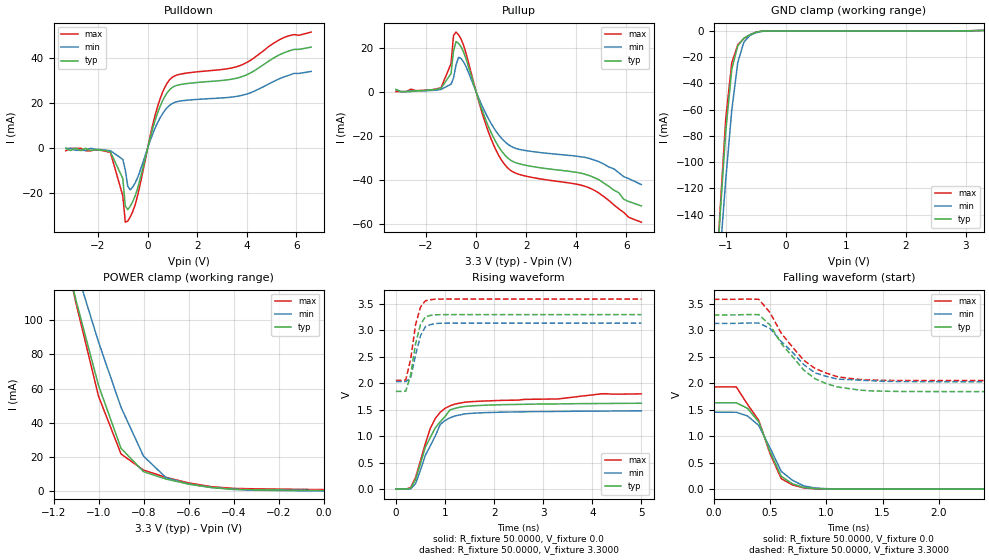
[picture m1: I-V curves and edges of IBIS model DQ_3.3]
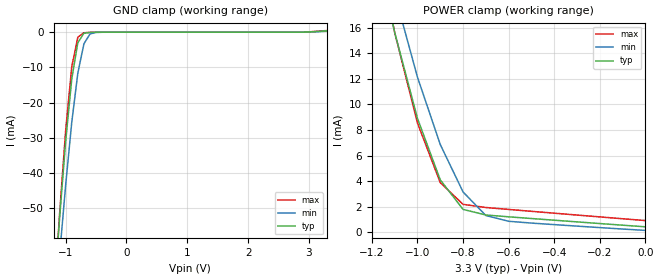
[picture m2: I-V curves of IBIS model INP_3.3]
|*** ISSI Synchronous Sram IBIS Model ***
[IBIS ver]	3.2
[File name]	is61lf204836b100tq.ibs
[File Rev]	1.0
[Date]	May 13,2013
[Notes]
|--- Version History --------------------------------
|1.0: prelimiary
[Disclaimer]	This information is for modeling purpose only
		and is not guaranteed
[Copyright]	INTEGRATED SILICON SOLUTION, INC. 2011
[Component]	IS61LF204836B_100TQ
[Manufacturer]	ISSI
[Package]
| variable   typ   min   max
R_pkg		105.88m			21.330m			174.58m
L_pkg		1.8700nH		0.5900nH		2.5200nH
C_pkg		0.2100pF		0.0600pF		0.2800pF
[Pin]  signal_name   model_name   R_pin   L_pin   C_pin
100   A   INP_3.3
99   A   INP_3.3
98   CEB   INP_3.3
97   CE2   INP_3.3
96   NC   NC
95   NC   NC
94   BWbB   INP_3.3
93   BWaB   INP_3.3
92   CE2B   INP_3.3
91   VDD   POWER
90   VSS   GND
89   CLK   INP_3.3
88   GWB   INP_3.3
87   BWEB   INP_3.3
86   OEB   INP_3.3
85   ADSCB   INP_3.3
84   ADSPB   INP_3.3
83   ADVB   INP_3.3
82   A   INP_3.3
81   A   INP_3.3
80   DQPb   DQ_3.3
79   DQb   DQ_3.3
78   DQb   DQ_3.3
77   VDDQ   POWER
76   VSS   GND
75   DQb   DQ_3.3
74   DQb   DQ_3.3
73   DQb   DQ_3.3
72   DQb   DQ_3.3
71   VSS   GND
70   VDDQ   POWER
69   DQb   DQ_3.3
68   DQb   DQ_3.3
67   VSS   GND
66   NC   NC
65   VDD   POWER
64   ZZ   INP_3.3
63   DQa   DQ_3.3
62   DQa   DQ_3.3
61   VDDQ   POWER
60   VSS   GND
59   DQa   DQ_3.3
58   DQa   DQ_3.3
57   DQa   DQ_3.3
56   DQa   DQ_3.3
55   VSS   GND
54   VDDQ   POWER
53   DQa   DQ_3.3
52   DQa   DQ_3.3
51   DQPa   DQ_3.3
50   A   INP_3.3
49   A   INP_3.3
48   A   INP_3.3
47   A   INP_3.3
46   A   INP_3.3
45   A   INP_3.3
44   A   INP_3.3
43   A   INP_3.3
42   A   INP_3.3
41   VDD   POWER
40   VSS   GND
39   A   INP_3.3
38   A   INP_3.3
37   A0   INP_3.3
36   A1   INP_3.3
35   A   INP_3.3
34   A   INP_3.3
33   A   INP_3.3
32   A   INP_3.3
31   MODE   INP_3.3
30   DQPd   DQ_3.3
29   DQd   DQ_3.3
28   DQd   DQ_3.3
27   VDDQ   POWER
26   VSS   GND
25   DQd   DQ_3.3
24   DQd   DQ_3.3
23   DQd   DQ_3.3
22   DQd   DQ_3.3
21   VSS   GND
20   VDDQ   POWER
19   DQd   DQ_3.3
18   DQd   DQ_3.3
17   VSS   GND
16   NC   NC
15   VDD   POWER
14   NC   NC
13   DQc   DQ_3.3
12   DQc   DQ_3.3
11   VDDQ   POWER
10   VSS   GND
9   DQc   DQ_3.3
8   DQc   DQ_3.3
7   DQc   DQ_3.3
6   DQc   DQ_3.3
5   VSS   GND
4   VDDQ   POWER
3   DQc   DQ_3.3
2   DQc   DQ_3.3
1   DQPc   DQ_3.3
| Models and submodels in the file (2): DQ_3.3 (3-state), INP_3.3 (Input)
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|   Model DQ_3.3
[Model]		DQ_3.3
Model_type	3-state
Polarity   Non-Inverting
Enable   Active-Low
Vmeas = 	0.7500V
Cref = 		5.0000pF
Rref = 		50.0000
Vref = 		1.2500V
C_comp   3.8290pF   3.3420pF   4.0300pF|
[Temperature Range]	  25.0000   100.0000   0.0
[Voltage Range]   3.3000V   3.1350V   3.6000V
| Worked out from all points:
|   slope of the pulldown table from 0 to 0.495 V, typ, clamps not added: 26.9 ohm
|   slope of the pullup table from 0 to 0.495 V, typ, clamps not added: 31.2 ohm
|   GND clamp passes 1 mA (typ) near -0.49 V on its own axis
|   POWER clamp passes 1 mA (typ) near -0.36 V on its own axis
|   rising waveform, R_fixture 50.0000, V_fixture 0.0: 20-80 % time 480ps typ, 408ps min, 447ps max; typ from 0 V to 1.62 V
|   rising waveform, R_fixture 50.0000, V_fixture 3.3000: 20-80 % time 178ps typ, 175ps min, 176ps max; typ from 1.84 V to 3.29 V
|   falling waveform, R_fixture 50.0000, V_fixture 0.0: 20-80 % time 195ps typ, 217ps min, 242ps max; typ from 1.63 V to 0 V
|   falling waveform, R_fixture 50.0000, V_fixture 3.3000: 20-80 % time 343ps typ, 315ps min, 335ps max; typ from 3.29 V to 1.84 V
[Pulldown]
|Voltage	  I(typ)   I(min)   I(max)
-3.3V     0A         0A         -1.1mA
-1.5V     -1.6mA     -1.08mA    -1.87mA
-1V       -13.48mA   -4.95mA    -21.15mA
-900mV    -25.69mA   -9.639mA   -32.88mA
-800mV    -27.28mA   -16.91mA   -32.39mA
-700mV    -25.77mA   -18.5mA    -30.54mA
-500mV    -21.13mA   -15.36mA   -25.04mA
400mV     15.63mA    11.35mA    18.49mA
900mV     26.18mA    19.21mA    30.66mA
3.7V      31.51mA    23.31mA    36.7mA
5.5V      42.5mA     31.77mA    49.28mA
6.6V      45mA       34.2mA     51.7mA
[Pullup]
|Voltage	  I(typ)   I(min)   I(max)
-3.2V     1mA        900uA      0A
-1.4V     1.5mA      990uA      1.76mA
-1V       8.19mA     3.366mA    12.71mA
-900mV    18.53mA    6.147mA    25.54mA
-800mV    22.75mA    12.11mA    27.08mA
-700mV    21.98mA    15.63mA    25.89mA
-500mV    18.06mA    13.53mA    21.17mA
400mV     -13.22mA   -10.27mA   -15.35mA
1.2V      -29.47mA   -23.28mA   -33.95mA
1.9V      -33.32mA   -26.66mA   -38.21mA
4.5V      -38.1mA    -30.33mA   -43.68mA
6.6V      -52mA      -42.3mA    -59.4mA
[GND_clamp]
|Voltage	  I(typ)   I(min)   I(max)
-3.3V     -1.893A    -1.626A    -2.116A
-1.2V     -220.2mA   -237.3mA   -225.5mA
-1.1V     -144.4mA   -173.5mA   -140.5mA
-1V       -76.37mA   -113.2mA   -66.76mA
-900mV    -29.2mA    -60.35mA   -24.24mA
-800mV    -11.34mA   -23.99mA   -10.52mA
-700mV    -5.573mA   -8.7mA     -5.892mA
-600mV    -2.907mA   -3.457mA   -3.011mA
-500mV    -1.075mA   -1.407mA   -999.8uA
-300mV    -9.492uA   -41.34uA   -5.052uA
3.3V      423.1uA    322.6uA    488.5uA
[POWER_clamp]
|Voltage	  I(typ)   I(min)   I(max)
-3.3V     1.424A     1.197A     1.604A
-1.2V     166.3mA    175.1mA    171.7mA
-1.1V     111.5mA    129.9mA    109.8mA
-1V       61.82mA    87.17mA    55.51mA
-900mV    25.05mA    49.03mA    21.74mA
-800mV    11.41mA    20.46mA    12.33mA
-700mV    7.064mA    7.924mA    8.056mA
-600mV    4.166mA    4.141mA    4.82mA
-500mV    2.143mA    2.162mA    2.625mA
-400mV    1.124mA    995.4uA    1.625mA
0V        423.1uA    141.8uA    910.6uA
[Ramp]
| variable   typ   min   max
dV/dt_r		0.9120/0.3809n   0.7302/0.3836n   1.1604/0.3404n
dV/dt_f		0.8694/0.3076n   0.7542/0.2869n   0.9210/0.3315n
R_load =	50.0000
[Rising Waveform]
R_fixture=	50.0000
V_fixture=	0.0
V_fixture_min=	0.0
V_fixture_max=	0.0
|time   V(typ)   V(min)   V(max)
0s        0V         533.2nV    0V
300ps     18.56mV    3.797mV    30.05mV
400ps     179mV      102.4mV    219.2mV
600ps     791.3mV    638.4mV    860.4mV
700ps     973.8mV    816.1mV    1.144V
900ps     1.268V     1.216V     1.448V
1.1ns     1.494V     1.344V     1.571V
1.4ns     1.559V     1.419V     1.639V
1.9ns     1.585V     1.445V     1.665V
5ns       1.62V      1.476V     1.797V
[Rising Waveform]
R_fixture=	50.0000
V_fixture=	3.3000
V_fixture_min=	3.1350
V_fixture_max=	3.6000
|time   V(typ)   V(min)   V(max)
0s        1.843V     2.029V     2.051V
200ps     1.847V     2.03V      2.057V
300ps     2.15V      2.093V     2.449V
400ps     2.742V     2.529V     3.102V
500ps     3.104V     2.892V     3.434V
600ps     3.25V      3.063V     3.552V
700ps     3.276V     3.103V     3.573V
800ps     3.288V     3.123V     3.583V
1ns       3.291V     3.131V     3.585V
5ns       3.292V     3.131V     3.585V
[Falling Waveform]
R_fixture=	50.0000
V_fixture=	0.0
V_fixture_min=	0.0
V_fixture_max=	0.0
|time   V(typ)   V(min)   V(max)
0s        1.632V     1.453V     1.932V
200ps     1.632V     1.452V     1.931V
300ps     1.527V     1.382V     1.602V
400ps     1.271V     1.204V     1.299V
500ps     710mV      779.4mV    671.9mV
600ps     241.6mV    335.5mV    197.9mV
700ps     100.8mV    166.6mV    80.02mV
800ps     32.06mV    61.86mV    23.86mV
1.2ns     262.2uV    1.546mV    276.4uV
5ns       29.31uV    38.72uV    18.07uV
[Falling Waveform]
R_fixture=	50.0000
V_fixture=	3.3000
V_fixture_min=	3.1350
V_fixture_max=	3.6000
|time   V(typ)   V(min)   V(max)
0s        3.292V     3.132V     3.586V
400ps     3.297V     3.139V     3.587V
500ps     3.102V     3.036V     3.335V
600ps     2.752V     2.791V     2.944V
800ps     2.249V     2.353V     2.434V
900ps     2.087V     2.196V     2.281V
1.1ns     1.931V     2.079V     2.123V
1.3ns     1.871V     2.058V     2.072V
1.6ns     1.847V     2.035V     2.054V
5ns       1.843V     2.029V     2.051V
|   Model INP_3.3
[Model]		INP_3.3
Model_type	Input
Polarity   Non-Inverting
Enable   Active-Low
Vinl = 		0.8000V
Vinh = 		2.0000V
C_comp   3.8290pF   3.3420pF   4.0300pF|
[Temperature Range]	  25.0000   100.0000   0.0
[Voltage Range]   3.3000V   3.1350V   3.6000V
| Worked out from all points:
|   GND clamp passes 1 mA (typ) near -0.73 V on its own axis
|   POWER clamp passes 1 mA (typ) near -0.45 V on its own axis
[GND_clamp]
|Voltage	  I(typ)   I(min)   I(max)
-3.3V     -664.2mA   -601mA     -729.6mA
-1.2V     -76.89mA   -84.89mA   -78.19mA
-1.1V     -52.83mA   -63.46mA   -51.66mA
-1V       -30.98mA   -43.42mA   -27.92mA
-900mV    -13.28mA   -25.61mA   -9.811mA
-800mV    -2.971mA   -11.61mA   -1.401mA
-700mV    -287uA     -3.303mA   -148.3uA
-600mV    -52.18uA   -480.7uA   -48.72uA
-500mV    -11.21uA   -45.78uA   -9.079uA
2.8V      415nA      176.2nA    769.3nA
3.3V      423.1uA    321.5uA    488.5uA
[POWER_clamp]
|Voltage	  I(typ)   I(min)   I(max)
-3.3V     318.3mA    284.6mA    350.6mA
-1.2V     23.85mA    26.22mA    24.49mA
-1.1V     15.64mA    18.66mA    15.62mA
-1V       8.908mA    12.13mA    8.545mA
-900mV    4.097mA    6.862mA    3.88mA
-800mV    1.786mA    3.15mA     2.181mA
-700mV    1.348mA    1.305mA    1.934mA
-600mV    1.205mA    856uA      1.783mA
0V        423.1uA    141.8uA    910.6uA
